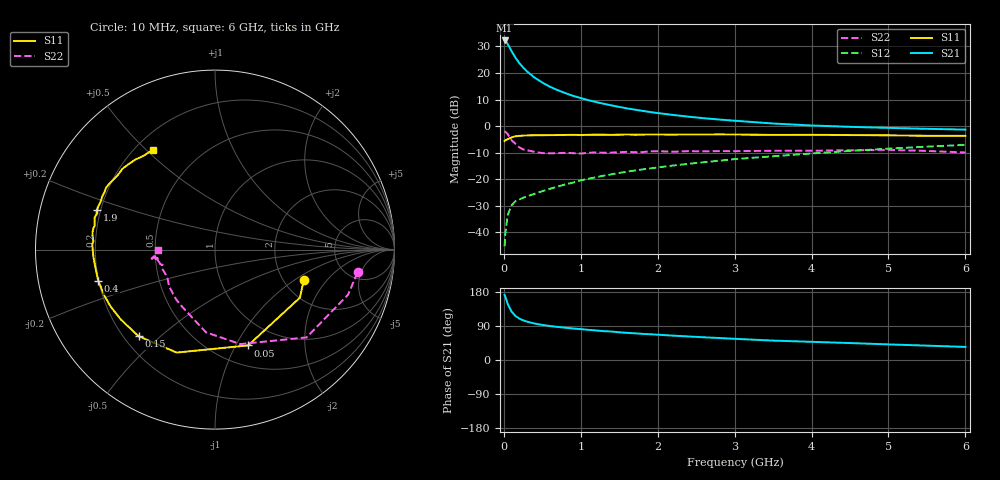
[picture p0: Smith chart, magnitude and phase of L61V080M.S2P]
!  INFINEON TECHNOLOGIES Small Signal Semiconductors
! BFR380L3 , Si-NPN RF-Transistor in TSLP-3-1
!  Vce=1 V,  Ic=80 mA
! Common Emitter S-Parameters:  07. March 2005
#  GHz  S  MA  R  50
! f  S11  S21  S12  S22
! GHz  Mag  Ang  Mag  Ang  Mag  Ang  Mag  Ang
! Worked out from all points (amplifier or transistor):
!   36 points, 10 MHz to 6 GHz, reference 50 ohm
!   highest |S21| = 32.2 dB at 10 MHz (marker M1)
!   |S21| within 3 dB of that: start of sweep to 81.41 MHz
!   unconditionally stable (mu >= 1): 773.1 MHz to end of sweep
!   at 250 MHz: K = 0.59, MSG = 24.5 dB, |S12| = -27.0 dB
!   at 1.4 GHz: K = 1.10, MAG = 11.0 dB, |S12| = -18.2 dB
!   at 6 GHz: K = 1.03, MAG = 1.8 dB, |S12| = -7.1 dB
!   S11 on the Smith chart (normalised r, x): 10 MHz: 2.55, -1.20; 50 MHz: 0.72, -1.12; 150 MHz: 0.26, -0.43; 400 MHz: 0.20, -0.13; 1.9 GHz: 0.19, +0.16; 6 GHz: 0.27, +0.52
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0.01  0.5229 -19.1  40.86 171.4  0.0055 63.9  0.8042 -9.1
0.02  0.5437 -29.5  39.99 166.5  0.0098 69.7  0.7828 -18.7
0.05  0.5648 -70.9  35.06 147.9  0.0211 60.2  0.7067 -43.8
0.1  0.6121 -110.4  25.81 127.9  0.0323 48.3  0.5451 -75.0
0.15  0.6435 -131.4  19.45 116.4  0.0384 44.1  0.4636 -96.2
0.2  0.6531 -143.1  15.38 109.5  0.0414 43.6  0.3993 -108.6
0.25  0.6625 -151.3  12.69 104.7  0.0448 43.5  0.3643 -121.3
0.3  0.6669 -156.8  10.7 101.3  0.0475 45.0  0.3514 -128.3
0.4  0.6734 -165.0  8.171 96.1  0.0532 48.0  0.3275 -141.5
0.5  0.6731 -170.2  6.597 92.6  0.0596 51.1  0.3106 -148.0
0.6  0.6757 -174.1  5.491 89.7  0.066 53.8  0.308 -152.7
0.7  0.6787 -176.7  4.744 87.3  0.0728 56.1  0.3095 -157.2
0.9  0.6844 177.4  3.706 83.2  0.0864 59.4  0.3095 -163.2
1.1  0.6853 174.0  3.071 79.6  0.1024 61.4  0.3152 -165.0
1.5  0.6891 166.8  2.291 73.1  0.1317 63.4  0.3231 -168.8
1.9  0.6938 161.4  1.842 68.0  0.1597 63.9  0.3348 -170.9
2.2  0.6913 157.5  1.62 64.3  0.181 63.6  0.3287 -171.4
2.6  0.6941 153.0  1.407 59.9  0.209 63.5  0.3343 -171.5
3.5  0.6823 142.2  1.118 51.2  0.2705 60.8  0.343 -172.7
4.5  0.6777 135.7  0.968 44.7  0.3409 58.1  0.3507 -172.3
5.5  0.6564 127.0  0.888 37.9  0.41 53.3  0.3407 -174.1
6  0.6558 121.9  0.858 34.5  0.4435 50.7  0.3186 -179.2
